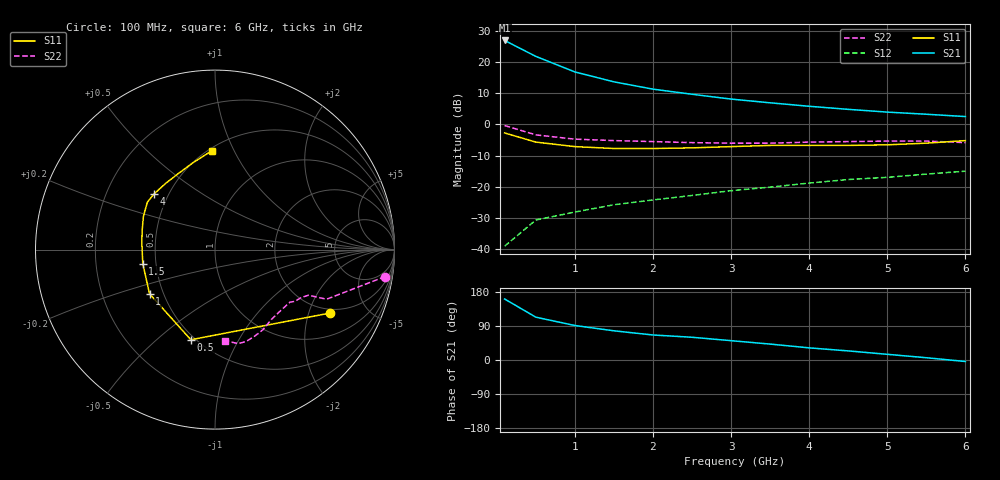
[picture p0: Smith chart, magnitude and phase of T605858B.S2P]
!AT-60585
!S-PARAMETERS at Vce=8V  Ic=10mA.  LAST UPDATED 07-21-92
# ghz s ma r 50
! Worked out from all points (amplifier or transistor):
!   13 points, 100 MHz to 6 GHz, reference 50 ohm
!   highest |S21| = 27.0 dB at 100 MHz (marker M1)
!   |S21| within 3 dB of that: start of sweep to 333.7 MHz
!   unconditionally stable (mu >= 1): 1.205 GHz to 5.661 GHz
!   at 1 GHz: K = 0.94, MSG = 22.5 dB, |S12| = -28.2 dB
!   at 3 GHz: K = 1.26, MAG = 11.6 dB, |S12| = -21.3 dB
!   at 6 GHz: K = 0.97, MSG = 8.8 dB, |S12| = -15.0 dB
!   S11 on the Smith chart (normalised r, x): 100 MHz: 1.82, -2.77; 500 MHz: 0.47, -0.65; 1 GHz: 0.42, -0.26; 1.5 GHz: 0.42, -0.08; 4 GHz: 0.42, +0.32; 6 GHz: 0.52, +0.82
0.1  0.73 -29.0  22.47 161.0  0.011 84.0  0.96 -9.0
0.5  0.52 -105.0  12.44 113.0  0.029 49.0  0.68 -24.0
1  0.44 -146.0  7 91.0  0.039 52.0  0.58 -26.0
1.5  0.41 -169.0  4.85 77.0  0.051 57.0  0.55 -29.0
2  0.41 174.0  3.7 66.0  0.061 58.0  0.53 -33.0
2.5  0.42 165.0  3.06 60.0  0.072 58.0  0.51 -35.0
3  0.44 155.0  2.56 51.0  0.086 65.0  0.5 -42.0
3.5  0.46 145.0  2.23 42.0  0.098 61.0  0.5 -51.0
4  0.46 138.0  1.96 32.0  0.114 59.0  0.52 -59.0
4.5  0.46 127.0  1.75 24.0  0.13 57.0  0.53 -65.0
5  0.47 116.0  1.58 15.0  0.141 52.0  0.54 -71.0
5.5  0.5 104.0  1.46 6.0  0.159 48.0  0.54 -76.0
6  0.55 92.0  1.34 -4.0  0.177 43.0  0.51 -84.0
